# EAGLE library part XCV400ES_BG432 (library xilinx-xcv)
xcv400es_bg432 edit this description Auto generated by make-symbol-device-package-bsdl.ulp Rev. 26 Source: xcv400es_bg432.bsd
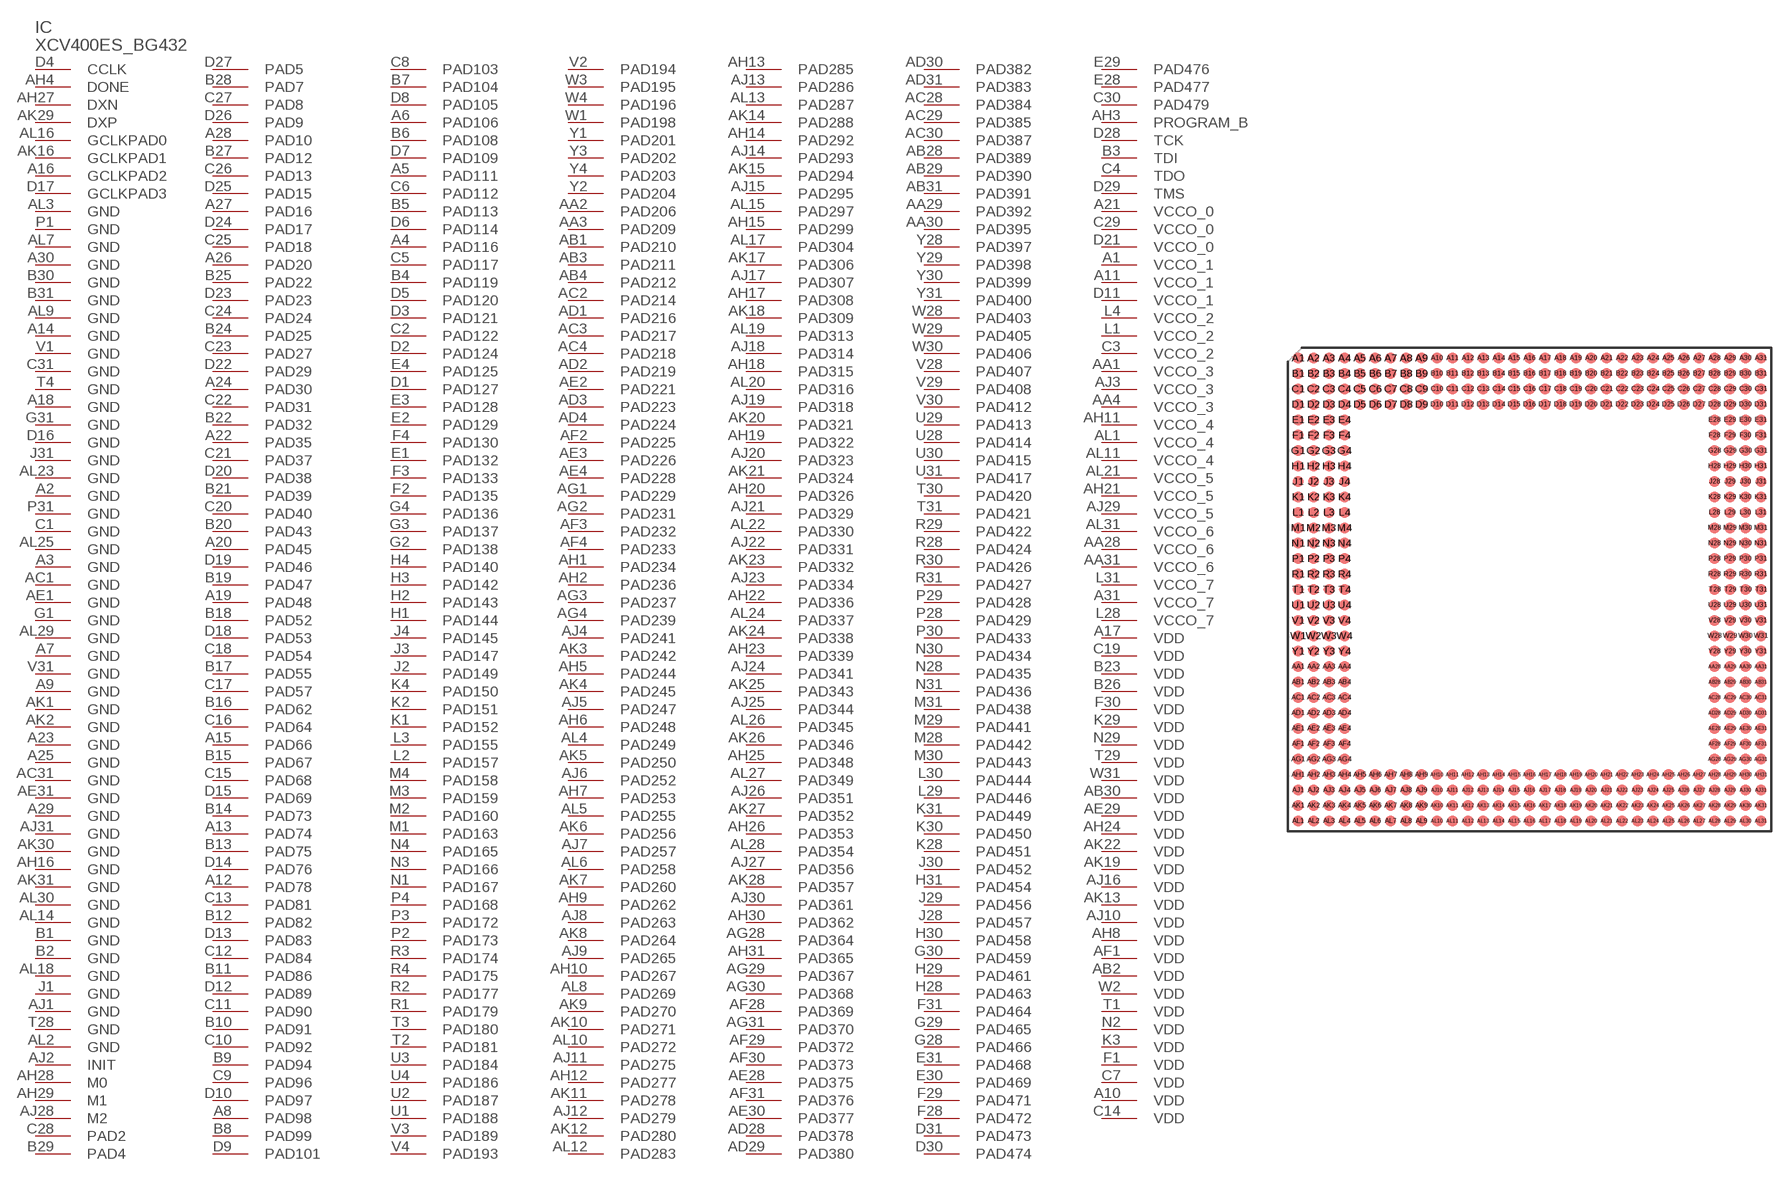
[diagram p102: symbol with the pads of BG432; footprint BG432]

Designator prefix IC

## XCV400ES_BG432 (OC_FARNELL: unknown; OC_NEWARK: unknown)  [BG432]
A1  VCCO_1  pwr
A2  GND  pwr
A3  GND  pwr
A4  PAD116
A5  PAD111
A6  PAD106
A7  GND  pwr
A8  PAD98
A9  GND  pwr
A10  VDD  pwr
A11  VCCO_1  pwr
A12  PAD78
A13  PAD74
A14  GND  pwr
A15  PAD66
A16  GCLKPAD2  in
A17  VDD  pwr
A18  GND  pwr
A19  PAD48
A20  PAD45
A21  VCCO_0  pwr
A22  PAD35
A23  GND  pwr
A24  PAD30
A25  GND  pwr
A26  PAD20
A27  PAD16
A28  PAD10
A29  GND  pwr
A30  GND  pwr
A31  VCCO_7  pwr
AA1  VCCO_3  pwr
AA2  PAD206
AA3  PAD209
AA4  VCCO_3  pwr
AA28  VCCO_6  pwr
AA29  PAD392
AA30  PAD395
AA31  VCCO_6  pwr
AB1  PAD210
AB2  VDD  pwr
AB3  PAD211
AB4  PAD212
AB28  PAD389
AB29  PAD390
AB30  VDD  pwr
AB31  PAD391
AC1  GND  pwr
AC2  PAD214
AC3  PAD217
AC4  PAD218
AC28  PAD384
AC29  PAD385
AC30  PAD387
AC31  GND  pwr
AD1  PAD216
AD2  PAD219
AD3  PAD223
AD4  PAD224
AD28  PAD378
AD29  PAD380
AD30  PAD382
AD31  PAD383
AE1  GND  pwr
AE2  PAD221
AE3  PAD226
AE4  PAD228
AE28  PAD375
AE29  VDD  pwr
AE30  PAD377
AE31  GND  pwr
AF1  VDD  pwr
AF2  PAD225
AF3  PAD232
AF4  PAD233
AF28  PAD369
AF29  PAD372
AF30  PAD373
AF31  PAD376
AG1  PAD229
AG2  PAD231
AG3  PAD237
AG4  PAD239
AG28  PAD364
AG29  PAD367
AG30  PAD368
AG31  PAD370
AH1  PAD234
AH2  PAD236
AH3  PROGRAM_B  in
AH4  DONE
AH5  PAD244
AH6  PAD248
AH7  PAD253
AH8  VDD  pwr
AH9  PAD262
AH10  PAD267
AH11  VCCO_4  pwr
AH12  PAD277
AH13  PAD285
AH14  PAD292
AH15  PAD299
AH16  GND  pwr
AH17  PAD308
AH18  PAD315
AH19  PAD322
AH20  PAD326
AH21  VCCO_5  pwr
AH22  PAD336
AH23  PAD339
AH24  VDD  pwr
AH25  PAD348
AH26  PAD353
AH27  DXN  pas
AH28  M0  in
AH29  M1  in
AH30  PAD362
AH31  PAD365
AJ1  GND  pwr
AJ2  INIT
AJ3  VCCO_3  pwr
AJ4  PAD241
AJ5  PAD247
AJ6  PAD252
AJ7  PAD257
AJ8  PAD263
AJ9  PAD265
AJ10  VDD  pwr
AJ11  PAD275
AJ12  PAD279
AJ13  PAD286
AJ14  PAD293
AJ15  PAD295
AJ16  VDD  pwr
AJ17  PAD307
AJ18  PAD314
AJ19  PAD318
AJ20  PAD323
AJ21  PAD329
AJ22  PAD331
AJ23  PAD334
AJ24  PAD341
AJ25  PAD344
AJ26  PAD351
AJ27  PAD356
AJ28  M2  in
AJ29  VCCO_5  pwr
AJ30  PAD361
AJ31  GND  pwr
AK1  GND  pwr
AK2  GND  pwr
AK3  PAD242
AK4  PAD245
AK5  PAD250
AK6  PAD256
AK7  PAD260
AK8  PAD264
AK9  PAD270
AK10  PAD271
AK11  PAD278
AK12  PAD280
AK13  VDD  pwr
AK14  PAD288
AK15  PAD294
AK16  GCLKPAD1  in
AK17  PAD306
AK18  PAD309
AK19  VDD  pwr
AK20  PAD321
AK21  PAD324
AK22  VDD  pwr
AK23  PAD332
AK24  PAD338
AK25  PAD343
AK26  PAD346
AK27  PAD352
AK28  PAD357
AK29  DXP  pas
AK30  GND  pwr
AK31  GND  pwr
AL1  VCCO_4  pwr
AL2  GND  pwr
AL3  GND  pwr
AL4  PAD249
AL5  PAD255
AL6  PAD258
AL7  GND  pwr
AL8  PAD269
AL9  GND  pwr
AL10  PAD272
AL11  VCCO_4  pwr
AL12  PAD283
AL13  PAD287
AL14  GND  pwr
AL15  PAD297
AL16  GCLKPAD0  in
AL17  PAD304
AL18  GND  pwr
AL19  PAD313
AL20  PAD316
AL21  VCCO_5  pwr
AL22  PAD330
AL23  GND  pwr
AL24  PAD337
AL25  GND  pwr
AL26  PAD345
AL27  PAD349
AL28  PAD354
AL29  GND  pwr
AL30  GND  pwr
AL31  VCCO_6  pwr
B1  GND  pwr
B2  GND  pwr
B3  TDI  in
B4  PAD119
B5  PAD113
B6  PAD108
B7  PAD104
B8  PAD99
B9  PAD94
B10  PAD91
B11  PAD86
B12  PAD82
B13  PAD75
B14  PAD73
B15  PAD67
B16  PAD62
B17  PAD55
B18  PAD52
B19  PAD47
B20  PAD43
B21  PAD39
B22  PAD32
B23  VDD  pwr
B24  PAD25
B25  PAD22
B26  VDD  pwr
B27  PAD12
B28  PAD7
B29  PAD4
B30  GND  pwr
B31  GND  pwr
C1  GND  pwr
C2  PAD122
C3  VCCO_2  pwr
C4  TDO  out
C5  PAD117
C6  PAD112
C7  VDD  pwr
C8  PAD103
C9  PAD96
C10  PAD92
C11  PAD90
C12  PAD84
C13  PAD81
C14  VDD  pwr
C15  PAD68
C16  PAD64
C17  PAD57
C18  PAD54
C19  VDD  pwr
C20  PAD40
C21  PAD37
C22  PAD31
C23  PAD27
C24  PAD24
C25  PAD18
C26  PAD13
C27  PAD8
C28  PAD2
C29  VCCO_0  pwr
C30  PAD479
C31  GND  pwr
D1  PAD127
D2  PAD124
D3  PAD121
D4  CCLK
D5  PAD120
D6  PAD114
D7  PAD109
D8  PAD105
D9  PAD101
D10  PAD97
D11  VCCO_1  pwr
D12  PAD89
D13  PAD83
D14  PAD76
D15  PAD69
D16  GND  pwr
D17  GCLKPAD3  in
D18  PAD53
D19  PAD46
D20  PAD38
D21  VCCO_0  pwr
D22  PAD29
D23  PAD23
D24  PAD17
D25  PAD15
D26  PAD9
D27  PAD5
D28  TCK  in
D29  TMS  in
D30  PAD474
D31  PAD473
E1  PAD132
E2  PAD129
E3  PAD128
E4  PAD125
E28  PAD477
E29  PAD476
E30  PAD469
E31  PAD468
F1  VDD  pwr
F2  PAD135
F3  PAD133
F4  PAD130
F28  PAD472
F29  PAD471
F30  VDD  pwr
F31  PAD464
G1  GND  pwr
G2  PAD138
G3  PAD137
G4  PAD136
G28  PAD466
G29  PAD465
G30  PAD459
G31  GND  pwr
H1  PAD144
H2  PAD143
H3  PAD142
H4  PAD140
H28  PAD463
H29  PAD461
H30  PAD458
H31  PAD454
J1  GND  pwr
J2  PAD149
J3  PAD147
J4  PAD145
J28  PAD457
J29  PAD456
J30  PAD452
J31  GND  pwr
K1  PAD152
K2  PAD151
K3  VDD  pwr
K4  PAD150
K28  PAD451
K29  VDD  pwr
K30  PAD450
K31  PAD449
L1  VCCO_2  pwr
L2  PAD157
L3  PAD155
L4  VCCO_2  pwr
L28  VCCO_7  pwr
L29  PAD446
L30  PAD444
L31  VCCO_7  pwr
M1  PAD163
M2  PAD160
M3  PAD159
M4  PAD158
M28  PAD442
M29  PAD441
M30  PAD443
M31  PAD438
N1  PAD167
N2  VDD  pwr
N3  PAD166
N4  PAD165
N28  PAD435
N29  VDD  pwr
N30  PAD434
N31  PAD436
P1  GND  pwr
P2  PAD173
P3  PAD172
P4  PAD168
P28  PAD429
P29  PAD428
P30  PAD433
P31  GND  pwr
R1  PAD179
R2  PAD177
R3  PAD174
R4  PAD175
R28  PAD424
R29  PAD422
R30  PAD426
R31  PAD427
T1  VDD  pwr
T2  PAD181
T3  PAD180
T4  GND  pwr
T28  GND  pwr
T29  VDD  pwr
T30  PAD420
T31  PAD421
U1  PAD188
U2  PAD187
U3  PAD184
U4  PAD186
U28  PAD414
U29  PAD413
U30  PAD415
U31  PAD417
V1  GND  pwr
V2  PAD194
V3  PAD189
V4  PAD193
V28  PAD407
V29  PAD408
V30  PAD412
V31  GND  pwr
W1  PAD198
W2  VDD  pwr
W3  PAD195
W4  PAD196
W28  PAD403
W29  PAD405
W30  PAD406
W31  VDD  pwr
Y1  PAD201
Y2  PAD204
Y3  PAD202
Y4  PAD203
Y28  PAD397
Y29  PAD398
Y30  PAD399
Y31  PAD400

## Footprint BG432 (pad centres in mm)
xcv300_bg432 edit this description Auto generated by make-symbol-device-package-bsdl.ulp Rev. 26 Source: xcv300_bg432.bsd
smd 0.9 x 0.9: A1 -19.05,19.05; A2 -17.78,19.05; A3 -16.51,19.05; A4 -15.24,19.05; A5 -13.97,19.05; A6 -12.7,19.05; A7 -11.43,19.05; A8 -10.16,19.05; A9 -8.89,19.05; A10 -7.62,19.05; A11 -6.35,19.05; A12 -5.08,19.05; A13 -3.81,19.05; A14 -2.54,19.05; A15 -1.27,19.05; A16 0,19.05; A17 1.27,19.05; A18 2.54,19.05; A19 3.81,19.05; A20 5.08,19.05; A21 6.35,19.05; A22 7.62,19.05; A23 8.89,19.05; A24 10.16,19.05; A25 11.43,19.05; A26 12.7,19.05; A27 13.97,19.05; A28 15.24,19.05; A29 16.51,19.05; A30 17.78,19.05; A31 19.05,19.05; AA1 -19.05,-6.35; AA2 -17.78,-6.35; AA3 -16.51,-6.35; AA4 -15.24,-6.35; AA28 15.24,-6.35; AA29 16.51,-6.35; AA30 17.78,-6.35; AA31 19.05,-6.35; AB1 -19.05,-7.62; AB2 -17.78,-7.62; AB3 -16.51,-7.62; AB4 -15.24,-7.62; AB28 15.24,-7.62; AB29 16.51,-7.62; AB30 17.78,-7.62; AB31 19.05,-7.62; AC1 -19.05,-8.89; AC2 -17.78,-8.89; AC3 -16.51,-8.89; AC4 -15.24,-8.89; AC28 15.24,-8.89; AC29 16.51,-8.89; AC30 17.78,-8.89; AC31 19.05,-8.89; AD1 -19.05,-10.16; AD2 -17.78,-10.16; AD3 -16.51,-10.16; AD4 -15.24,-10.16; AD28 15.24,-10.16; AD29 16.51,-10.16; AD30 17.78,-10.16; AD31 19.05,-10.16; AE1 -19.05,-11.43; AE2 -17.78,-11.43; AE3 -16.51,-11.43; AE4 -15.24,-11.43; AE28 15.24,-11.43; AE29 16.51,-11.43; AE30 17.78,-11.43; AE31 19.05,-11.43; AF1 -19.05,-12.7; AF2 -17.78,-12.7; AF3 -16.51,-12.7; AF4 -15.24,-12.7; AF28 15.24,-12.7; AF29 16.51,-12.7; AF30 17.78,-12.7; AF31 19.05,-12.7; AG1 -19.05,-13.97; AG2 -17.78,-13.97; AG3 -16.51,-13.97; AG4 -15.24,-13.97; AG28 15.24,-13.97; AG29 16.51,-13.97; AG30 17.78,-13.97; AG31 19.05,-13.97; AH1 -19.05,-15.24; AH2 -17.78,-15.24; AH3 -16.51,-15.24; AH4 -15.24,-15.24; AH5 -13.97,-15.24; AH6 -12.7,-15.24; AH7 -11.43,-15.24; AH8 -10.16,-15.24; AH9 -8.89,-15.24; AH10 -7.62,-15.24; AH11 -6.35,-15.24; AH12 -5.08,-15.24; AH13 -3.81,-15.24; AH14 -2.54,-15.24; AH15 -1.27,-15.24; AH16 0,-15.24; AH17 1.27,-15.24; AH18 2.54,-15.24; AH19 3.81,-15.24; AH20 5.08,-15.24; AH21 6.35,-15.24; AH22 7.62,-15.24; AH23 8.89,-15.24; AH24 10.16,-15.24; AH25 11.43,-15.24; AH26 12.7,-15.24; AH27 13.97,-15.24; AH28 15.24,-15.24; AH29 16.51,-15.24; AH30 17.78,-15.24; AH31 19.05,-15.24; AJ1 -19.05,-16.51; AJ2 -17.78,-16.51; AJ3 -16.51,-16.51; AJ4 -15.24,-16.51; AJ5 -13.97,-16.51; AJ6 -12.7,-16.51; AJ7 -11.43,-16.51; AJ8 -10.16,-16.51; AJ9 -8.89,-16.51; AJ10 -7.62,-16.51; AJ11 -6.35,-16.51; AJ12 -5.08,-16.51; AJ13 -3.81,-16.51; AJ14 -2.54,-16.51; AJ15 -1.27,-16.51; AJ16 0,-16.51; AJ17 1.27,-16.51; AJ18 2.54,-16.51; AJ19 3.81,-16.51; AJ20 5.08,-16.51; AJ21 6.35,-16.51; AJ22 7.62,-16.51; AJ23 8.89,-16.51; AJ24 10.16,-16.51; AJ25 11.43,-16.51; AJ26 12.7,-16.51; AJ27 13.97,-16.51; AJ28 15.24,-16.51; AJ29 16.51,-16.51; AJ30 17.78,-16.51; AJ31 19.05,-16.51; AK1 -19.05,-17.78; AK2 -17.78,-17.78; AK3 -16.51,-17.78; AK4 -15.24,-17.78; AK5 -13.97,-17.78; AK6 -12.7,-17.78; AK7 -11.43,-17.78; AK8 -10.16,-17.78; AK9 -8.89,-17.78; AK10 -7.62,-17.78; AK11 -6.35,-17.78; AK12 -5.08,-17.78; AK13 -3.81,-17.78; AK14 -2.54,-17.78; AK15 -1.27,-17.78; AK16 0,-17.78; AK17 1.27,-17.78; AK18 2.54,-17.78; AK19 3.81,-17.78; AK20 5.08,-17.78; AK21 6.35,-17.78; AK22 7.62,-17.78; AK23 8.89,-17.78; AK24 10.16,-17.78; AK25 11.43,-17.78; AK26 12.7,-17.78; AK27 13.97,-17.78; AK28 15.24,-17.78; AK29 16.51,-17.78; AK30 17.78,-17.78; AK31 19.05,-17.78; AL1 -19.05,-19.05; AL2 -17.78,-19.05; AL3 -16.51,-19.05; AL4 -15.24,-19.05; AL5 -13.97,-19.05; AL6 -12.7,-19.05; AL7 -11.43,-19.05; AL8 -10.16,-19.05; AL9 -8.89,-19.05; AL10 -7.62,-19.05; AL11 -6.35,-19.05; AL12 -5.08,-19.05; AL13 -3.81,-19.05; AL14 -2.54,-19.05; AL15 -1.27,-19.05; AL16 0,-19.05; AL17 1.27,-19.05; AL18 2.54,-19.05; AL19 3.81,-19.05; AL20 5.08,-19.05; AL21 6.35,-19.05; AL22 7.62,-19.05; AL23 8.89,-19.05; AL24 10.16,-19.05; AL25 11.43,-19.05; AL26 12.7,-19.05; AL27 13.97,-19.05; AL28 15.24,-19.05; AL29 16.51,-19.05; AL30 17.78,-19.05; AL31 19.05,-19.05; B1 -19.05,17.78; B2 -17.78,17.78; B3 -16.51,17.78; B4 -15.24,17.78; B5 -13.97,17.78; B6 -12.7,17.78; B7 -11.43,17.78; B8 -10.16,17.78; B9 -8.89,17.78; B10 -7.62,17.78; B11 -6.35,17.78; B12 -5.08,17.78; B13 -3.81,17.78; B14 -2.54,17.78; B15 -1.27,17.78; B16 0,17.78; B17 1.27,17.78; B18 2.54,17.78; B19 3.81,17.78; B20 5.08,17.78; B21 6.35,17.78; B22 7.62,17.78; B23 8.89,17.78; B24 10.16,17.78; B25 11.43,17.78; B26 12.7,17.78; B27 13.97,17.78; B28 15.24,17.78; B29 16.51,17.78; B30 17.78,17.78; B31 19.05,17.78; C1 -19.05,16.51; C2 -17.78,16.51; C3 -16.51,16.51; C4 -15.24,16.51; C5 -13.97,16.51; C6 -12.7,16.51; C7 -11.43,16.51; C8 -10.16,16.51; C9 -8.89,16.51; C10 -7.62,16.51; C11 -6.35,16.51; C12 -5.08,16.51; C13 -3.81,16.51; C14 -2.54,16.51; C15 -1.27,16.51; C16 0,16.51; C17 1.27,16.51; C18 2.54,16.51; C19 3.81,16.51; C20 5.08,16.51; C21 6.35,16.51; C22 7.62,16.51; C23 8.89,16.51; C24 10.16,16.51; C25 11.43,16.51; C26 12.7,16.51; C27 13.97,16.51; C28 15.24,16.51; C29 16.51,16.51; C30 17.78,16.51; C31 19.05,16.51; D1 -19.05,15.24; D2 -17.78,15.24; D3 -16.51,15.24; D4 -15.24,15.24; D5 -13.97,15.24; D6 -12.7,15.24; D7 -11.43,15.24; D8 -10.16,15.24; D9 -8.89,15.24; D10 -7.62,15.24; D11 -6.35,15.24; D12 -5.08,15.24; D13 -3.81,15.24; D14 -2.54,15.24; D15 -1.27,15.24; D16 0,15.24; D17 1.27,15.24; D18 2.54,15.24; D19 3.81,15.24; D20 5.08,15.24; D21 6.35,15.24; D22 7.62,15.24; D23 8.89,15.24; D24 10.16,15.24; D25 11.43,15.24; D26 12.7,15.24; D27 13.97,15.24; D28 15.24,15.24; D29 16.51,15.24; D30 17.78,15.24; D31 19.05,15.24; E1 -19.05,13.97; E2 -17.78,13.97; E3 -16.51,13.97; E4 -15.24,13.97; E28 15.24,13.97; E29 16.51,13.97; E30 17.78,13.97; E31 19.05,13.97; F1 -19.05,12.7; F2 -17.78,12.7; F3 -16.51,12.7; F4 -15.24,12.7; F28 15.24,12.7; F29 16.51,12.7; F30 17.78,12.7; F31 19.05,12.7; G1 -19.05,11.43; G2 -17.78,11.43; G3 -16.51,11.43; G4 -15.24,11.43; G28 15.24,11.43; G29 16.51,11.43; G30 17.78,11.43; G31 19.05,11.43; H1 -19.05,10.16; H2 -17.78,10.16; H3 -16.51,10.16; H4 -15.24,10.16; H28 15.24,10.16; H29 16.51,10.16; H30 17.78,10.16; H31 19.05,10.16; J1 -19.05,8.89; J2 -17.78,8.89; J3 -16.51,8.89; J4 -15.24,8.89; J28 15.24,8.89; J29 16.51,8.89; J30 17.78,8.89; J31 19.05,8.89; K1 -19.05,7.62; K2 -17.78,7.62; K3 -16.51,7.62; K4 -15.24,7.62; K28 15.24,7.62; K29 16.51,7.62; K30 17.78,7.62; K31 19.05,7.62; L1 -19.05,6.35; L2 -17.78,6.35; L3 -16.51,6.35; L4 -15.24,6.35; L28 15.24,6.35; L29 16.51,6.35; L30 17.78,6.35; L31 19.05,6.35; M1 -19.05,5.08; M2 -17.78,5.08; M3 -16.51,5.08; M4 -15.24,5.08; M28 15.24,5.08; M29 16.51,5.08; M30 17.78,5.08; M31 19.05,5.08; N1 -19.05,3.81; N2 -17.78,3.81; N3 -16.51,3.81; N4 -15.24,3.81; N28 15.24,3.81; N29 16.51,3.81; N30 17.78,3.81; N31 19.05,3.81; P1 -19.05,2.54; P2 -17.78,2.54; P3 -16.51,2.54; P4 -15.24,2.54; P28 15.24,2.54; P29 16.51,2.54; P30 17.78,2.54; P31 19.05,2.54; R1 -19.05,1.27; R2 -17.78,1.27; R3 -16.51,1.27; R4 -15.24,1.27; R28 15.24,1.27; R29 16.51,1.27; R30 17.78,1.27; R31 19.05,1.27; T1 -19.05,0; T2 -17.78,0; T3 -16.51,0; T4 -15.24,0; T28 15.24,0; T29 16.51,0; T30 17.78,0; T31 19.05,0; U1 -19.05,-1.27; U2 -17.78,-1.27; U3 -16.51,-1.27; U4 -15.24,-1.27; U28 15.24,-1.27; U29 16.51,-1.27; U30 17.78,-1.27; U31 19.05,-1.27; V1 -19.05,-2.54; V2 -17.78,-2.54; V3 -16.51,-2.54; V4 -15.24,-2.54; V28 15.24,-2.54; V29 16.51,-2.54; V30 17.78,-2.54; V31 19.05,-2.54; W1 -19.05,-3.81; W2 -17.78,-3.81; W3 -16.51,-3.81; W4 -15.24,-3.81; W28 15.24,-3.81; W29 16.51,-3.81; W30 17.78,-3.81; W31 19.05,-3.81; Y1 -19.05,-5.08; Y2 -17.78,-5.08; Y3 -16.51,-5.08; Y4 -15.24,-5.08; Y28 15.24,-5.08; Y29 16.51,-5.08; Y30 17.78,-5.08; Y31 19.05,-5.08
